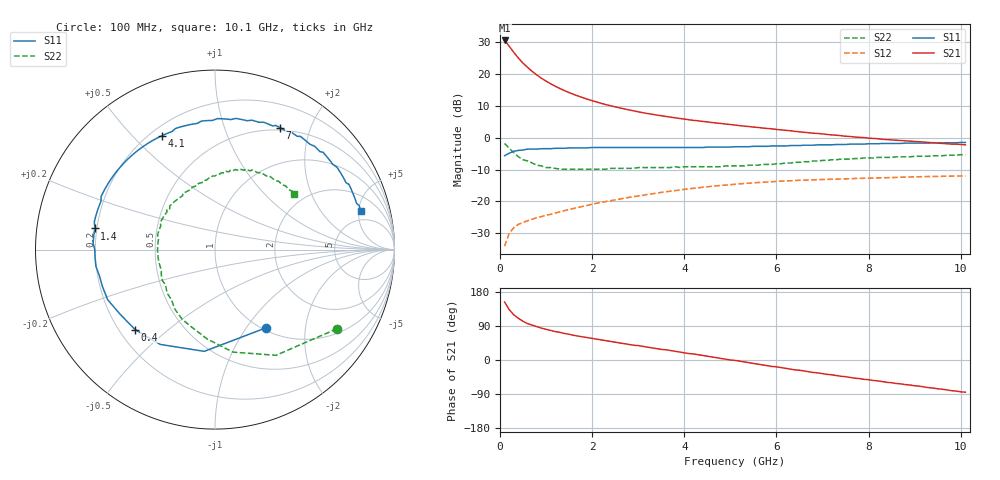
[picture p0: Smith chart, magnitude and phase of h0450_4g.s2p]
!HBFP-0450
!S and NOISE PARAMETERS at Vce=4V  Ic=35mA.  LAST UPDATED  09-04-98
# GHZ S MA R  50
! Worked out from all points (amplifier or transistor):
!   101 points, 100 MHz to 10.1 GHz, reference 50 ohm
!   highest |S21| = 30.4 dB at 100 MHz (marker M1)
!   |S21| within 3 dB of that: start of sweep to 261.7 MHz
!   unconditionally stable (mu >= 1): 2.302 GHz to end of sweep
!   at 1.7 GHz: K = 0.92, MSG = 17.4 dB, |S12| = -21.8 dB
!   at 5.1 GHz: K = 1.09, MAG = 7.5 dB, |S12| = -14.6 dB
!   at 10.1 GHz: K = 1.06, MAG = 3.4 dB, |S12| = -12.0 dB
!   lowest NFmin = 1.57 dB at 1.8 GHz
!   S11 on the Smith chart (normalised r, x): 100 MHz: 1.04, -1.24; 400 MHz: 0.26, -0.39; 1.4 GHz: 0.19, +0.08; 4.1 GHz: 0.24, +0.61; 7 GHz: 0.47, +1.56; 10.1 GHz: 3.55, +5.25
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0.1  0.52 -57.0  33.09 153.0  0.02 59.0  0.81 -33.0
0.2  0.57 -96.0  26.88 133.0  0.032 50.0  0.68 -60.0
0.3  0.61 -120.0  21.51 119.0  0.039 43.0  0.58 -80.0
0.4  0.63 -135.0  17.51 110.0  0.044 40.0  0.5 -95.0
0.5  0.64 -146.0  14.59 102.0  0.047 38.0  0.45 -107.0
0.6  0.66 -155.0  12.52 96.0  0.05 36.0  0.43 -115.0
0.7  0.66 -162.0  10.83 92.0  0.053 36.0  0.4 -124.0
0.8  0.66 -167.0  9.52 88.0  0.056 36.0  0.37 -131.0
0.9  0.67 -172.0  8.47 84.0  0.058 36.0  0.36 -138.0
1  0.67 -176.0  7.64 81.0  0.061 37.0  0.34 -144.0
1.2  0.68 177.0  6.35 75.0  0.066 37.0  0.33 -155.0
1.4  0.68 170.0  5.43 70.0  0.072 37.0  0.32 -164.0
1.8  0.69 160.0  4.2 61.0  0.084 37.0  0.32 -178.0
2.2  0.7 151.0  3.43 53.0  0.097 35.0  0.32 171.0
2.5  0.7 144.0  3.02 47.0  0.106 33.0  0.33 164.0
3.5  0.7 126.0  2.2 28.0  0.139 24.0  0.34 145.0
4.1  0.7 115.0  1.9 17.0  0.158 17.0  0.35 134.0
5.1  0.72 96.0  1.57 -1.0  0.186 3.0  0.36 116.0
6.8  0.76 65.0  1.17 -33.0  0.218 -21.0  0.43 85.0
7  0.77 62.0  1.14 -36.0  0.221 -24.0  0.44 82.0
8.5  0.81 39.0  0.92 -60.0  0.237 -44.0  0.49 61.0
10.1  0.84 15.0  0.77 -85.0  0.251 -66.0  0.54 35.0
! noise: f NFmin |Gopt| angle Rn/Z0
1.8  1.57  0.56  -155  0.08
2  1.6  0.55  -153  0.09
2.5  1.73  0.58  -142  0.13
3.5  1.98  0.62  -125  0.26
4  2.16  0.64  -115  0.39
5  2.44  0.67  -95  0.72
5.5  2.58  0.7  -85  1
7  3  0.75  -58  2.06
8  3.29  0.79  -42  3.02
10  3.84  0.82  -13  4.95
